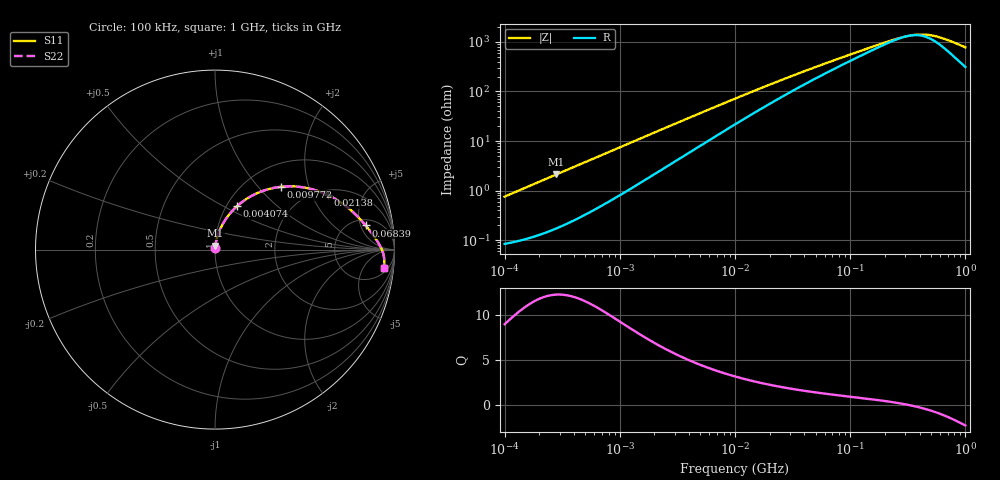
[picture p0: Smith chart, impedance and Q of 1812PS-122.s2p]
# MHz S MA R 50
!Freq  MagS11  AngS11  MagS21  AngS21  MagS12  AngS12  MagS22  AngS22
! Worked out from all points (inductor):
!   801 points, 100 kHz to 1 GHz, reference 50 ohm
!   read as one part in series: L = 1.2 uH near 104.7 kHz
!   highest Q = 12.2 at 281.8 kHz (marker M1), where L = 1.19 uH
!   self-resonance near 318.2 MHz
!   S11 on the Smith chart (normalised r, x): 100 kHz: 1.00, +0.02; 4.074 MHz: 1.12, +0.59; 9.772 MHz: 1.42, +1.34; 21.38 MHz: 2.23, +2.65; 68.39 MHz: 6.32, +6.14; 1 GHz: 7, -14
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0.1  0.007563 83.2  0.9991 -0.4  0.9991 -0.4  0.007563 83.2
0.2818383  0.02118 84.1  0.998 -1.2  0.998 -1.2  0.02118 84.1
0.4677351  0.03502 83.1  0.9964 -2.0  0.9964 -2.0  0.03502 83.1
1.071519  0.07924 79.1  0.9881 -4.5  0.9881 -4.5  0.07924 79.1
2.162719  0.1552 72.6  0.9649 -8.8  0.9649 -8.8  0.1552 72.6
3.019952  0.2106 68.0  0.9416 -12.0  0.9416 -12.0  0.2106 68.0
4.073803  0.2728 63.0  0.909 -15.5  0.909 -15.5  0.2728 63.0
6.16595  0.3773 54.5  0.839 -21.5  0.839 -21.5  0.3773 54.5
9.772372  0.507 43.6  0.7233 -28.9  0.7233 -28.9  0.507 43.6
10  0.5135 43.1  0.7166 -29.3  0.7166 -29.3  0.5135 43.1
14.28894  0.609 34.5  0.6059 -34.7  0.6059 -34.7  0.609 34.5
21.37962  0.6993 25.7  0.4784 -39.3  0.4784 -39.3  0.6993 25.7
31.26079  0.7642 18.8  0.3706 -41.7  0.3706 -41.7  0.7642 18.8
46.77351  0.8149 13.1  0.2773 -41.9  0.2773 -41.9  0.8149 13.1
68.39116  0.8503 9.1  0.2093 -40.0  0.2093 -40.0  0.8503 9.1
216.2719  0.9161 1.7  0.08883 -18.3  0.08883 -18.3  0.9161 1.7
331.1311  0.9308 -0.2  0.06925 2.4  0.06925 2.4  0.9308 -0.2
389.0451  0.9353 -0.9  0.0665 12.9  0.0665 12.9  0.9353 -0.9
451.8559  0.9389 -1.6  0.06694 23.3  0.06694 23.3  0.9389 -1.6
524.8075  0.9419 -2.4  0.07055 33.3  0.07055 33.3  0.9419 -2.4
616.595  0.9443 -3.2  0.07804 42.9  0.07804 42.9  0.9443 -3.2
1000  0.9449 -6.4  0.1216 59.9  0.1216 59.9  0.9449 -6.4
